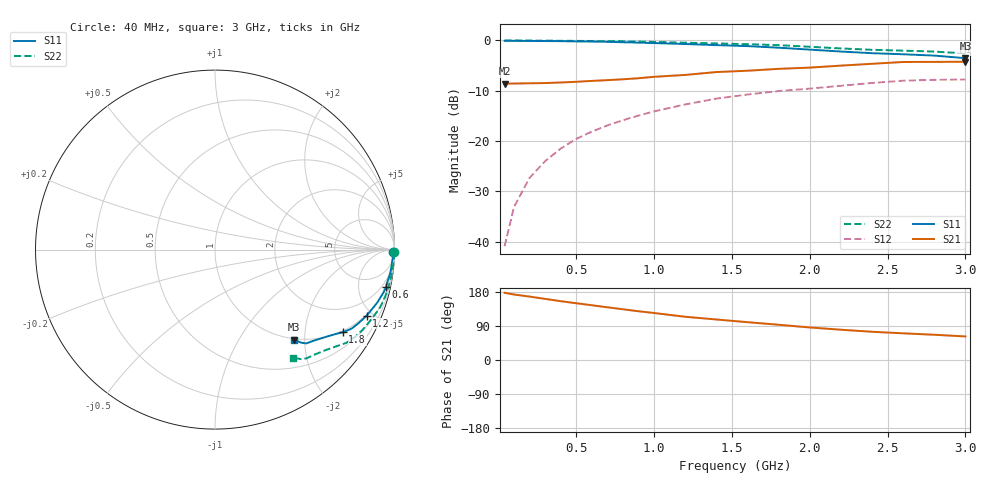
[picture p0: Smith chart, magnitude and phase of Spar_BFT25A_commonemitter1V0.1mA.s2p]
! Filename:  BFT25AA.S2P  Version:  2.0
! NXP part #: BFT25A  Date: Aug 1990
! Bias condition: Vce=1V, Ic=0.1mA
#  MHz  S  MA  R  50
! Freq  S11  S21  S12  S22  !GUM [dB]
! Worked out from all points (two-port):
!   21 points, 40 MHz to 3 GHz, reference 50 ohm
!   highest |S21| = -4.24 dB at 3 GHz (marker M1); lowest = -8.6 dB at 40 MHz (marker M2)
!   |S21| within 3 dB of the highest: 997.7 MHz to end of sweep
!   lowest |S11| = -3.5 dB at 3 GHz (marker M3), VSWR 5.01, Z = 48.9 - j88.5 ohm
!   |S11| at or under -10 dB: nowhere
!   |S22| runs from -2.6 to 0.0 dB; largest |S21 - S12| = 0.37
!   S11 on the Smith chart (normalised r, x): 40 MHz: open; 600 MHz: 1.11, -9.23; 1.2 GHz: 0.94, -4.62; 1.8 GHz: 0.96, -3.12; 3 GHz: 0.98, -1.77
40  0.993 -0.9  0.372 177.4  0.009 86.4  1 -0.9
100  0.992 -2.1  0.373 172.8  0.022 88.4  0.999 -2.2
200  0.989 -4.2  0.375 167.4  0.043 86.0  0.997 -4.4
300  0.987 -6.3  0.377 161.3  0.063 84.2  0.995 -6.6
400  0.984 -8.2  0.382 155.2  0.084 82.4  0.993 -8.9
500  0.978 -10.2  0.388 149.8  0.105 80.7  0.99 -11.0
600  0.975 -12.2  0.396 144.5  0.124 79.1  0.987 -13.1
700  0.969 -14.2  0.403 139.1  0.143 77.3  0.984 -15.1
800  0.96 -16.0  0.411 133.9  0.161 75.5  0.98 -17.1
900  0.952 -17.9  0.421 128.6  0.179 73.6  0.975 -19.1
1000  0.942 -19.6  0.435 124.0  0.197 71.9  0.967 -21.0
1200  0.922 -23.5  0.454 114.1  0.231 67.8  0.95 -24.9
1400  0.899 -27.1  0.485 106.9  0.264 64.5  0.935 -28.8
1600  0.879 -30.1  0.5 99.8  0.29 61.3  0.918 -32.1
1800  0.847 -32.9  0.522 93.0  0.314 58.3  0.898 -35.3
2000  0.811 -35.8  0.537 85.9  0.332 54.3  0.865 -38.5
2200  0.776 -39.3  0.562 79.9  0.354 50.4  0.833 -42.2
2400  0.747 -42.9  0.586 74.5  0.378 47.2  0.807 -46.4
2600  0.729 -45.8  0.611 70.4  0.398 44.6  0.792 -49.9
2800  0.707 -47.2  0.612 66.6  0.406 42.5  0.775 -51.9
3000  0.667 -48.9  0.614 62.2  0.409 40.4  0.743 -54.2
